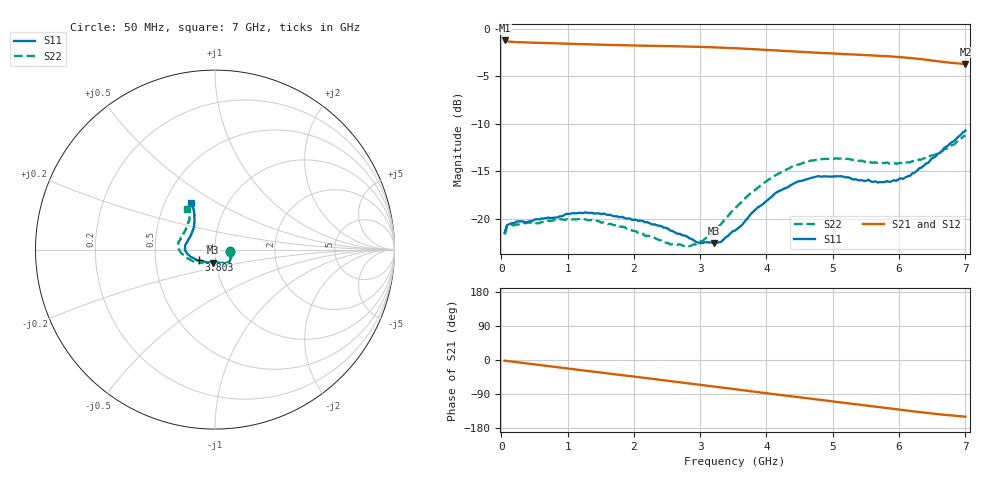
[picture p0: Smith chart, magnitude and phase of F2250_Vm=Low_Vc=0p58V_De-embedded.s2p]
! Integrated Device Technology
! Corporate Headquarters
! 6024 Silver Creek Valley Road
! San Jose, CA 95138  USA
! Phone:  1-408-284-8200
! Toll Free:  1-800-223-1366
! Webpage:  http://www.idt.com/
! Timing and RF Division
! 515 Groton Road, Suite 102
! Westford, MA 01886-6024
! Device:  F2250
! Description: Voltage Variable RF Attenuator
! Frequency:  50.0 -  6000.00 MHz
! Package:  3x3 mm Thin QFN Plastic Package: 16 pin
! Ports:  2 RF, 3 DC
!  Pin  1  = GND
!  Pin  2  = NC
!  Pin  3  = RF1  = Port 1
!  Pin  4  = NC
!  Pin  5  = GND
!  Pin  6  = GND
!  Pin  7  = GND
!  Pin  8  = GND
!  Pin  9  = NC
!  Pin 10  = RF2  = Port 2
!  Pin 11  = NC
!  Pin 12  = GND
!  Pin 13  = GND
!  Pin 14  = VCNTRL
!  Pin 15  = VDD
!  Pin 16  = VMODE
! Vcntrl:  0.580 Volts
! Vmode:  +0.000 Volts
! Vdd:  +3.30  Volts
! Current:  1.134 mA
! Data:  The device was measured on a the F2250 evaluation board which has
!  individual transmission lines to the RF pins.  Data was collected
!  using a calibrated network analyzer.  The evaluation board was
!  de-embedded using a TRL calibration technique.
!  The reference plane is the edge of the package pin.
! Misc:  SN 10
!  Action Tracker AT0258
! Date Measured:  2014-11-26
! Date:  2015-10-15  MJV
! Note:
!  Integrated Device Technology supplies this data as a sample of measured
!  data at the package pin for this product.  Your particular data for this
!  product may vary.
!  Data was taken at 25 degrees C.
!  Integrated Device Technology reserves the right to change this data at anytime.
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# GHz S dB R 50
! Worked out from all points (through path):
!   201 points, 50 MHz to 7 GHz, reference 50 ohm
!   highest |S21| = -1.21 dB at 50 MHz (marker M1); lowest = -3.7 dB at 7 GHz (marker M2)
!   group delay of S21, straight-line fit = 60.1 ps
!   lowest |S11| = -22.6 dB at 3.212 GHz (marker M3), VSWR 1.16, Z = 48.4 - j7.15 ohm
!   |S11| at or under -10 dB: start of sweep to end of sweep
!   |S22| runs from -22.9 to -11.2 dB; largest |S21 - S12| = 0.00046
!   S11 on the Smith chart (normalised r, x): 50 MHz: 1.18, -0.02; 3.803 GHz: 0.83, -0.10; 7 GHz: 0.68, +0.39
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0.05  -21.45 -6.5  -1.21 -1.8  -1.21 -1.8  -21.66 -7.5
0.08475  -20.68 -6.6  -1.30 -2.5  -1.30 -2.5  -20.87 -7.2
0.15425  -20.47 -8.6  -1.35 -4.0  -1.35 -4.0  -20.65 -9.0
0.71025  -19.86 -29.8  -1.49 -16.2  -1.49 -16.2  -20.19 -33.5
1.2315  -19.39 -45.4  -1.61 -27.4  -1.61 -27.4  -20.07 -53.2
1.75275  -19.75 -52.2  -1.70 -38.5  -1.70 -38.5  -20.64 -62.9
2.37825  -20.71 -54.9  -1.79 -51.8  -1.79 -51.8  -22.22 -71.2
2.552  -21.23 -58.1  -1.81 -55.6  -1.81 -55.6  -22.71 -77.1
2.83  -22.02 -68.7  -1.86 -61.7  -1.86 -61.7  -22.88 -92.6
3.0385  -22.54 -83.7  -1.90 -66.3  -1.90 -66.3  -22.31 -108.1
3.21225  -22.59 -98.3  -1.94 -70.2  -1.94 -70.2  -21.28 -121.1
3.3165  -22.42 -109.5  -1.96 -72.5  -1.96 -72.5  -20.54 -128.0
3.525  -21.23 -127.4  -2.03 -77.2  -2.03 -77.2  -18.91 -140.1
3.803  -19.23 -146.7  -2.13 -83.3  -2.13 -83.3  -17.08 -153.1
4.1505  -17.20 -161.8  -2.27 -91.0  -2.27 -91.0  -15.35 -167.1
4.7065  -15.63 -178.2  -2.48 -103.0  -2.48 -103.0  -13.86 178.6
5.15825  -15.56 170.7  -2.64 -112.7  -2.64 -112.7  -13.62 168.9
5.85325  -16.10 146.8  -2.89 -127.6  -2.89 -127.6  -14.18 153.1
6.166  -15.45 134.6  -3.05 -134.4  -3.06 -134.4  -14.05 144.0
6.444  -14.08 124.8  -3.26 -140.2  -3.26 -140.2  -13.53 134.5
6.82625  -11.83 117.9  -3.58 -146.9  -3.58 -146.9  -12.17 126.2
7  -10.71 116.9  -3.70 -149.6  -3.70 -149.6  -11.21 124.6
